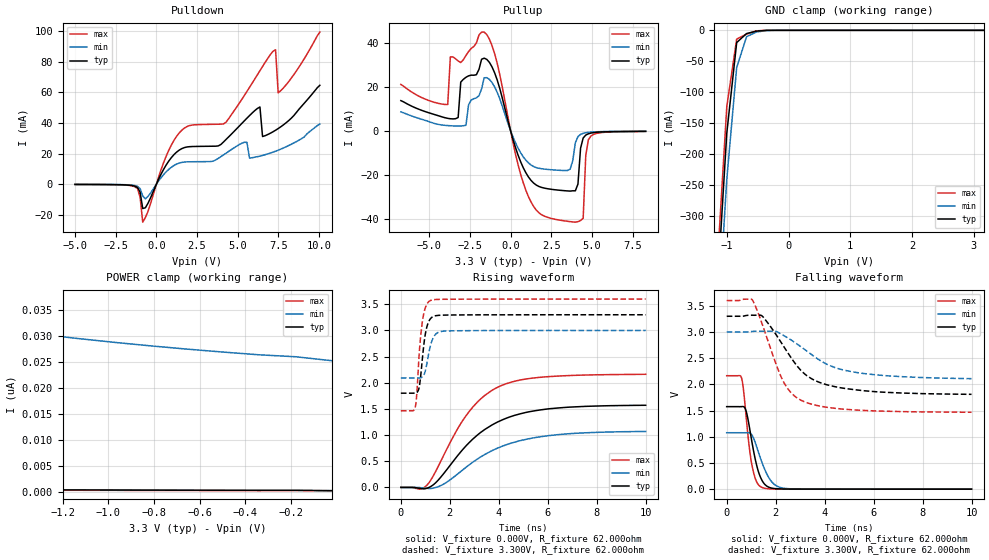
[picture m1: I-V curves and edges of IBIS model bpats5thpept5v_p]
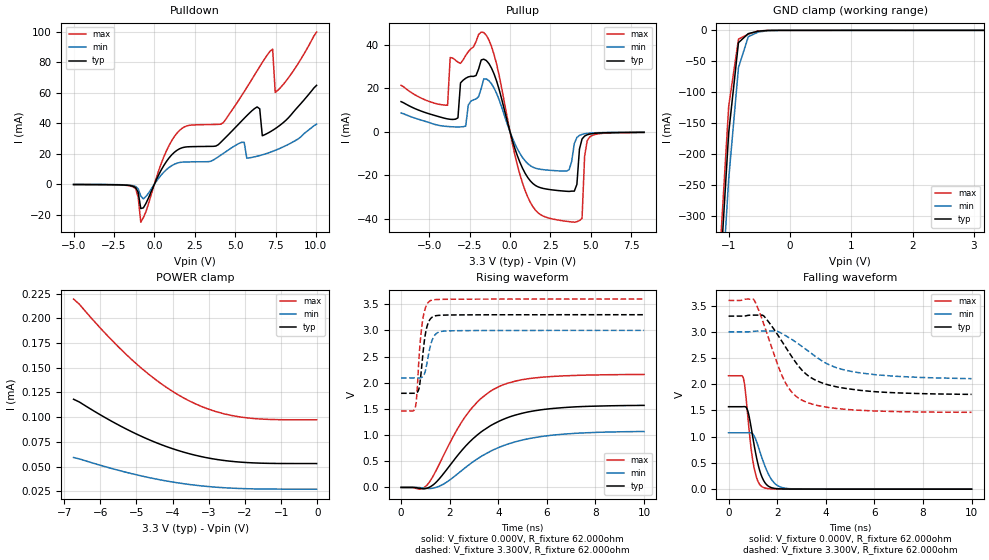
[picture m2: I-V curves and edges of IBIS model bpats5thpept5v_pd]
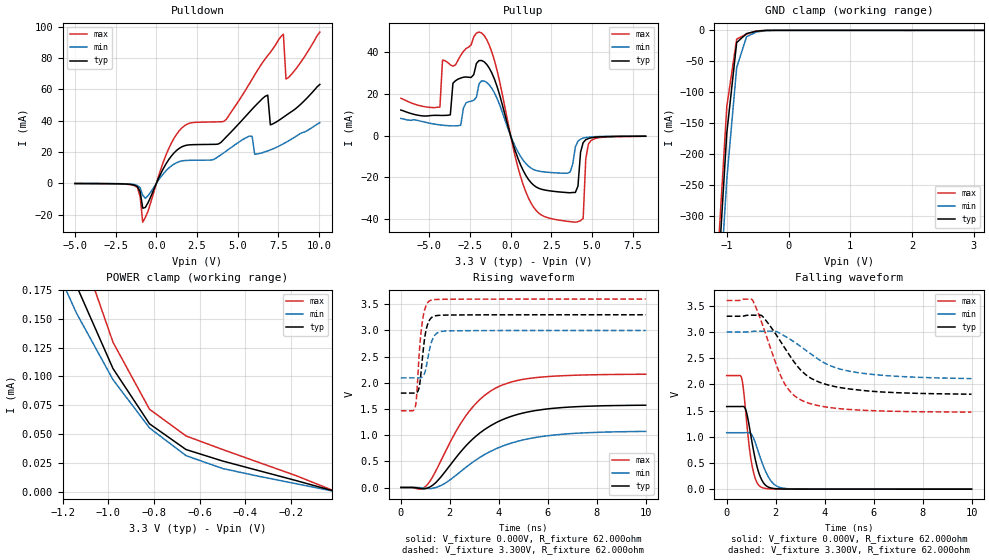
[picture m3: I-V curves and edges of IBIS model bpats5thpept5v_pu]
[IBIS Ver]  4.0
[File Name]  lpc176x.ibs
[File Rev]  1.0
[Date]   Tue Jul 28 17:01:21 PDT 2009
[Source]   Package model from Ansoft Q3D Extractor 7.1.1
[Notes]   IO models Rev 0.20 IBIS Model Design Automation Generation
[Copyright] NXP Semiconductors 2009. All rights reserved.
|   LPC1768 / 1766 / 1765 / 1764 IBIS Model
[Disclaimer]
| NXP Semiconductors warrants and represents that the IBIS models
| identified herein are owned by NXP Semiconductors (NXP).  The
| models provided are not warranted as fully representing all of the
| operating characteristics and specifications of the semiconductor
| products to which the models relate.  Moreover, unless there is a
| signed, written agreement to the contrary, these models are furnished
| on an "as is" basis without support or warranty of any kind, either
| expressed or implied, regarding the use thereof, and NXP
| specifically disclaims all implied warranties of merchantability and
| fitness of the models for any purpose.
| NXP does not assume any liability arising out of the application
| or use of these IBIS models including infringement of patents and
| copyrights, nor does NXP convey any license under its patents and
| copyrights or the rights of others.
| NXP provides IBIS models as a service to our customers.  You and
| your company shall not distribute, convey, sell, or give these models
| to anyone else without receiving prior written permission from
| NXP.
[Define Package Model]  LQFP100
[Manufacturer]  NXP Semiconductors
[OEM]  NXP
[Description]  LQFP100
|Sim freq : 100HMz
|Date : 7/28/09
[Number Of Pins]  100
[Pin Numbers]
1   | 1 = lead1
2   | 2 = lead2
3   | 3 = lead3
4   | 4 = lead4
5   | 5 = lead5
6   | 6 = lead6
7   | 7 = lead7
8   | 8 = lead8
9   | 9 = lead9
10   | 10 = lead10
11   | 11 = lead11
12   | 12 = lead12
13   | 13 = lead13
14   | 14 = lead14
15   | 15 = lead15
16   | 16 = lead16
17   | 17 = lead17
18   | 18 = lead18
19   | 19 = lead19
20   | 20 = lead20
21   | 21 = lead21
22   | 22 = lead22
23   | 23 = lead23
24   | 24 = lead24
25   | 25 = lead25
26   | 26 = lead26
27   | 27 = lead27
28   | 28 = lead28
29   | 29 = lead29
30   | 30 = lead30
31   | 31 = lead31
32   | 32 = lead32
33   | 33 = lead33
34   | 34 = lead34
35   | 35 = lead35
36   | 36 = lead36
37   | 37 = lead37
38   | 38 = lead38
39   | 39 = lead39
40   | 40 = lead40
41   | 41 = lead41
42   | 42 = lead42
43   | 43 = lead43
44   | 44 = lead44
45   | 45 = lead45
46   | 46 = lead46
47   | 47 = lead47
48   | 48 = lead48
49   | 49 = lead49
50   | 50 = lead50
51   | 51 = lead51
52   | 52 = lead52
53   | 53 = lead53
54   | 54 = lead54
55   | 55 = lead55
56   | 56 = lead56
57   | 57 = lead57
58   | 58 = lead58
59   | 59 = lead59
60   | 60 = lead60
61   | 61 = lead61
62   | 62 = lead62
63   | 63 = lead63
64   | 64 = lead64
65   | 65 = lead65
66   | 66 = lead66
67   | 67 = lead67
68   | 68 = lead68
69   | 69 = lead69
70   | 70 = lead70
71   | 71 = lead71
72   | 72 = lead72
73   | 73 = lead73
74   | 74 = lead74
75   | 75 = lead75
76   | 76 = lead76
77   | 77 = lead77
78   | 78 = lead78
79   | 79 = lead79
80   | 80 = lead80
81   | 81 = lead81
82   | 82 = lead82
83   | 83 = lead83
84   | 84 = lead84
85   | 85 = lead85
86   | 86 = lead86
87   | 87 = lead87
88   | 88 = lead88
89   | 89 = lead89
90   | 90 = lead90
91   | 91 = lead91
92   | 92 = lead92
93   | 93 = lead93
94   | 94 = lead94
95   | 95 = lead95
96   | 96 = lead96
97   | 97 = lead97
98   | 98 = lead98
99   | 99 = lead99
100   | 100 = lead100
[Model Data]
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[End Model Data]
[End Package Model]
[Component]   lpc176x
[Manufacturer]  NXP
[Package]
|   typ   min   max
R_pkg   0   0   0  |Values included in package model
L_pkg   0   0   0  |Values included in package model
C_pkg   0   0   0  |Values included in package model
[Package Model]  LQFP100
| (Pin and IO model definitions)
| IMPORTANT NOTES:
| The lpc176x GPIO pins, excluding the I2C and USB, have programmable input
| configurations. For this reason, three models are supplied for those basic
| padcells. Each model is identified by a unique suffix code at the end of
| the modelname:
| _p=plain input, _pd=pulldown enabled, _pu=pullup enabled
| The model_name for each of the GPIO pins in the [Pin] table below reflects
| the default state of that pin on power up (input with pullup enabled).
| The user may modify the model_name for a specific P#.# pin if that pin's
| input configuration is programmed differently from the default in the
| actual application. However, the model_names for all other pins are
| non-configurable and should not be altered.
| All GPIO padcells have 5ns slew rate control when operated as outputs,
| unless otherwise noted.
[Pin]   signal_name   model_name   | comments
1   TDO   bpts5ptpht5v_p   | 3-state output only
2   TDI   bpts5ptpht5v_pu   | In only
3   TMS   bpts5ptpht5v_pu   |
4   TRST_N   bpts5ptpht5v_pu   | In only
5   TCK   bpts5ptpht5v_p   | In only
6   P0.26   bpats5thpept5v_pu |
7   P0.25   bpats5thpept5v_pu |
8   P0.24   bpats5thpept5v_pu |
9   P0.23   bpats5thpept5v_pu |
10   VddA   POWER
11   VssA   GND
12   VREFP   POWER
13   Vdd   POWER
14   RSTOUTN   bpts5ptpht5v_pu   | Output only
15   VREFN   GND
16   RTCX1   NC
17   NRESET   bpts5ptpht5v_pu   | In only
18   RTCX2   NC
19   VBAT   POWER
20   P1.31   bpats5thpept5v_pu |
21   P1.30   bpats5thpept5v_pu |
22   X1   NC
23   X2   NC
24   P0.28   iic3m4sdat5v_400k | I2C padcell
25   P0.27   iic3m4sdat5v_400k | I2C padcell
26   P3.26   bpts5ptpht5v_pu   |
27   P3.25   bpts5ptpht5v_pu   |
28   Vdd   POWER
29   P0.29   usb11f1_iop_hs   | USB padcell
30   P0.30   usb11f1_iom_hs   | USB padcell
31   Vss   GND
32   P1.18   bpts5ptpht5v_pu   |
33   P1.19   bpts5ptpht5v_pu   |
34   P1.20   bpts5ptpht5v_pu   |
35   P1.21   bpts5ptpht5v_pu   |
36   P1.22   bpts5ptpht5v_pu   |
37   P1.23   bpts5ptpht5v_pu   |
38   P1.24   bpts5ptpht5v_pu   |
39   P1.25   bpts5ptpht5v_pu   |
40   P1.26   bpts5ptpht5v_pu   |
41   Vss   GND
42   Vdd   POWER
43   P1.27   bpts5ptpht5v_pu   |
44   P1.28   bpts5ptpht5v_pu   |
45   P1.29   bpts5ptpht5v_pu   |
46   P0.0   bpts5ptpht5v_pu   |
47   P0.1   bpts5ptpht5v_pu   |
48   P0.10   bpts5ptpht5v_pu   |
49   P0.11   bpts5ptpht5v_pu   |
50   P2.13   bpts5ptpht5v_pu   |
51   P2.12   bpts5ptpht5v_pu   |
52   P2.11   bpts5ptpht5v_pu   |
53   P2.10   bpts5ptpht5v_pu   |
54   Vdd   POWER
55   Vss   GND
56   P0.22   bpts5ptpht5v_pu   |
57   P0.21   bpts5ptpht5v_pu   |
58   P0.20   bpts5ptpht5v_pu   |
59   P0.19   bpts5ptpht5v_pu   |
60   P0.18   bpts5ptpht5v_pu   |
61   P0.17   bpts5ptpht5v_pu   |
62   P0.15   bpts5ptpht5v_pu   |
63   P0.16   bpts5ptpht5v_pu   |
64   P2.9   bpts5ptpht5v_pu   |
65   P2.8   bpts5ptpht5v_pu   |
66   P2.7   bpts5ptpht5v_pu   |
67   P2.6   bpts5ptpht5v_pu   |
68   P2.5   bpts5ptpht5v_pu   |
69   P2.4   bpts5ptpht5v_pu   |
70   P2.3   bpts5ptpht5v_pu   |
71   Vdd   POWER
72   Vss   GND
73   P2.2   bpts5ptpht5v_pu   |
74   P2.1   bpts5ptpht5v_pu   |
75   P2.0   bpts5ptpht5v_pu   |
76   P0.9   bpts5ptpht5v_pu   |
77   P0.8   bpts5ptpht5v_pu   |
78   P0.7   bpts5ptpht5v_pu   |
79   P0.6   bpts5ptpht5v_pu   |
80   P0.5   bpts5ptpht5v_pu   |
81   P0.4   bpts5ptpht5v_pu   |
82   P4.28   bpts5ptpht5v_pu   |
83   Vss   GND
84   Vdd   POWER
85   P4.29   bpts5ptpht5v_pu   |
86   P1.17   bpts5ptpht5v_pu   |
87   P1.16   bpts5ptpht5v_pu   |
88   P1.15   bpts5ptpht5v_pu   |
89   P1.14   bpts5ptpht5v_pu   |
90   P1.10   bpts5ptpht5v_pu   |
91   P1.9   bpts5ptpht5v_pu   |
92   P1.8   bpts5ptpht5v_pu   |
93   P1.4   bpts5ptpht5v_pu   |
94   P1.1   bpts5ptpht5v_pu   |
95   P1.0   bpts5ptpht5v_pu   |
96   Vdd   POWER
97   Vss   GND
98   P0.2   bpts5ptpht5v_pu   |
99   P0.3   bpts5ptpht5v_pu   |
100   RTCK   bpts5ptpht5v_pu   |
| Models and submodels in the file (9): bpats5thpept5v_p (I/O), bpats5thpept5v_pd (I/O), bpats5thpept5v_pu (I/O), bpts5ptpht5v_p (I/O), bpts5ptpht5v_pd (I/O), bpts5ptpht5v_pu (I/O), iic3m4sdat5v_400k (I/O_open_drain), usb11f1_iom_hs (I/O), usb11f1_iop_hs (I/O)
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| bpats5thpept5v
|   Bidirectional Pad 3v3
|   CMOS
|   Characterized at Core 1.8V and I/O 3.3V
| Plain input Mode (p1=0, p2=1)
[Model]   bpats5thpept5v_p | of bpats5thpept5v
Model_type   I/O
Polarity   Non-Inverting
Enable   Active-Low
|  Reciever Thresholds
Vinl   = 0.54V
Vinh   = 1.26V
| AC Test Load Conditions
Vref   = 0
Cref   = 1.2e-11
Rref   = 1000000000
Vmeas   = 0.9
| [Process Range]   typical   min   max
| C_comp edge width   400.000ps   400.000ps   400.000ps
| C_comp Tstrobe   40.000fs   40.000fs   40.000fs
C_comp   2.539pF   2.402pF   2.679pF
[Temperature Range]   25   125   -40
[Voltage Range]   3.30V   3.00V   3.60V
[GND Clamp Reference]   0.00V   0.00V   0.00V
[Pulldown Reference]   0.00V   0.00V   0.00V
[POWER Clamp Reference]   3.30V   3.00V   3.60V
[Pullup Reference]   3.30V   3.00V   3.60V
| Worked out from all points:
|   slope of the pulldown table from 0 to 0.495 V, typ, clamps not added: 46.5 ohm
|   slope of the pullup table from 0 to 0.495 V, typ, clamps not added: 41.9 ohm
|   GND clamp passes 1 mA (typ) near -0.48 V on its own axis
|   rising waveform, V_fixture 0.000V, R_fixture 62.000ohm: 20-80 % time 2.15ns typ, 2.37ns min, 1.8ns max; typ from 0 V to 1.57 V
|   falling waveform, V_fixture 0.000V, R_fixture 62.000ohm: 20-80 % time 411ps typ, 539ps min, 319ps max; typ from 1.57 V to 0 V
|   rising waveform, V_fixture 3.300V, R_fixture 62.000ohm: 20-80 % time 225ps typ, 260ps min, 215ps max; typ from 1.8 V to 3.3 V
|   falling waveform, V_fixture 3.300V, R_fixture 62.000ohm: 20-80 % time 1.53ns typ, 1.95ns min, 1.1ns max; typ from 3.3 V to 1.81 V
[GND Clamp]
| ref voltage   0.00V   0.00V   0.00V
|   Voltage   I(typ)   I(min)   I(max)
-5V       -7.933A    -7.953A    -7.929A
-1.16V    -429.6mA   -501mA     -389.4mA
-1V       -166.1mA   -240.8mA   -123.1mA
-840mV    -19.82mA   -60.19mA   -14.18mA
-680mV    -5.225mA   -10.28mA   -6.152mA
-520mV    -1.304mA   -2.7mA     -818.1uA
-200mV    -132.3nA   -9.731uA   -2.769nA
3.16V     216.3pA    26.32nA    148.8pA
[Power Clamp]   | Vtable = Vcc - Vpad
| ref voltage   3.30V   3.00V   3.60V
|   Voltage   I(typ)   I(min)   I(max)
-6.74V    1.379nA    125.5nA    723.8pA
-4.66V    863pA      70.57nA    560.5pA
-2.42V    509.5pA    38.28nA    388.3pA
-2.26V    489.9pA    36.89nA    376pA
-2.1V     470.8pA    35.59nA    363.8pA
-1.78V    434.1pA    33.27nA    339.4pA
-1.62V    416.5pA    32.24nA    327.2pA
-1.3V     382.5pA    30.41nA    302.8pA
-820mV    334.3pA    28.18nA    266.3pA
-340mV    288.9pA    26.43nA    229.9pA
-180mV    281.7pA    26.06nA    265.9pA
-20mV     233pA      25.29nA    176.8pA
[Pulldown]
| ref voltage   0.00V   0.00V   0.00V
|   Voltage   I(typ)   I(min)   I(max)
-5V       -187.5uA   -145.8uA   -211.8uA
-1.32V    -1.32mA    -939.5uA   -1.723mA
-1V       -5.324mA   -2.961mA   -8.618mA
-840mV    -15.95mA   -7.735mA   -24.89mA
1.4V      22.26mA    13.79mA    33.48mA
4.28V     29.27mA    20.27mA    40.55mA
5.56V     43.15mA    27.33mA    60.63mA
6.36V     50.49mA    18.36mA    74.24mA
6.52V     31.16mA    18.79mA    76.97mA
7.32V     35.27mA    21.55mA    87.95mA
7.48V     36.36mA    22.22mA    59.78mA
10.04V    64.68mA    39.32mA    99.49mA
[Pullup]   | Vtable = Vcc - Vpad
| ref voltage   3.30V   3.00V   3.60V
|   Voltage   I(typ)   I(min)   I(max)
-6.74V    13.67mA    8.53mA     21.02mA
-3.86V    5.598mA    2.307mA    11.88mA
-3.7V     5.416mA    2.227mA    33.56mA
-2.74V    24.29mA    2.441mA    34.22mA
-1.62V    32.99mA    24.07mA    44.83mA
940mV     -19.18mA   -13.46mA   -27.14mA
2.86V     -27.01mA   -17.98mA   -40.52mA
3.98V     -27.37mA   -5.511mA   -41.66mA
4.46V     -3.36mA    -1.235mA   -39.89mA
4.62V     -2.02mA    -961.6uA   -11.27mA
4.94V     -1.105mA   -662.3uA   -2.417mA
8.3V      -310.5uA   -276.1uA   -365.1uA
[Ramp]
R_load   = 62.000ohm
|   dV/dt(typ)   dV/dt(min)   dV/dt(max)
dV/dt_r   720.631mV/2.205ns   482.682mV/2.365ns   1.049V/2.035ns
dV/dt_f   674.653mV/1.565ns   397.637mV/1.940ns   1.038V/1.245ns
[Rising Waveform]  | cubic spline decimation from 2001 points
V_fixture   = 0.000V
R_fixture   = 62.000ohm
|   Time   V(typ)   V(min)   V(max)
0s        2.482nV    412.2nV    1.344nV
765ps     -17.12mV   -3.168mV   -33.52mV
1.06ns    -16.23mV   -17.53mV   40.55mV
1.715ns   244.2mV    54.65mV    580.5mV
2.665ns   795.4mV    385.7mV    1.372V
3.255ns   1.049V     581mV      1.689V
3.95ns    1.25V      750.6mV    1.914V
4.895ns   1.409V     895.8mV    2.055V
6.08ns    1.504V     991.8mV    2.119V
10ns      1.57V      1.07V      2.162V
[Falling Waveform]  | cubic spline decimation from 2001 points
V_fixture   = 0.000V
R_fixture   = 62.000ohm
|   Time   V(typ)   V(min)   V(max)
0s        1.575V     1.077V     2.165V
610ps     1.576V     1.077V     2.118V
680ps     1.576V     1.076V     1.921V
790ps     1.496V     1.077V     1.406V
1.025ns   917.9mV    1.038V     476.3mV
1.205ns   493mV      837.1mV    157.9mV
1.445ns   165.7mV    505.2mV    32.07mV
1.885ns   16.15mV    117.4mV    4.029mV
2.4ns     2.893mV    14.38mV    1.574mV
10ns      49.83uV    118.5uV    23.14uV
[Rising Waveform]  | cubic spline decimation from 2001 points
V_fixture   = 3.300V
V_fixture_min = 3.000V
V_fixture_max = 3.600V
R_fixture   = 62.000ohm
|   Time   V(typ)   V(min)   V(max)
0s        1.801V     2.092V     1.464V
585ps     1.801V     2.093V     1.532V
640ps     1.809V     2.093V     1.718V
755ps     1.929V     2.092V     2.589V
885ps     2.487V     2.116V     3.188V
1.03ns    3.005V     2.289V     3.47V
1.21ns    3.225V     2.71V      3.572V
1.41ns    3.281V     2.923V     3.591V
1.82ns    3.294V     2.989V     3.596V
10ns      3.3V       3V         3.6V
[Falling Waveform]  | cubic spline decimation from 2001 points
V_fixture   = 3.300V
V_fixture_min = 3.000V
V_fixture_max = 3.600V
R_fixture   = 62.000ohm
|   Time   V(typ)   V(min)   V(max)
0s        3.3V       3V         3.6V
1.04ns    3.32V      3.009V     3.616V
1.45ns    3.304V     3.014V     3.151V
2.045ns   2.929V     3.004V     2.35V
2.325ns   2.727V     2.933V     2.045V
2.66ns    2.488V     2.839V     1.826V
3.1ns     2.235V     2.695V     1.683V
4.145ns   1.986V     2.371V     1.559V
5.13ns    1.904V     2.24V      1.515V
10ns      1.81V      2.109V     1.468V
| bpats5thpept5v
|   Bidirectional Pad 3v3
|   CMOS
|   Characterized at Core 1.8V and I/O 3.3V
| Pull Down Mode (p1=1, p2=1)
[Model]   bpats5thpept5v_pd | of bpats5thpept5v
Model_type   I/O
Polarity   Non-Inverting
Enable   Active-Low
|  Reciever Thresholds
Vinl   = 0.54V
Vinh   = 1.26V
| AC Test Load Conditions
Vref   = 0
Cref   = 1.2e-11
Rref   = 1000000000
Vmeas   = 0.9
| [Process Range]   typical   min   max
| C_comp edge width   400.000ps   400.000ps   400.000ps
| C_comp Tstrobe   40.000fs   40.000fs   40.000fs
C_comp   2.538pF   2.399pF   2.678pF
[Temperature Range]   25   125   -40
[Voltage Range]   3.30V   3.00V   3.60V
[GND Clamp Reference]   0.00V   0.00V   0.00V
[Pulldown Reference]   0.00V   0.00V   0.00V
[POWER Clamp Reference]   3.30V   3.00V   3.60V
[Pullup Reference]   3.30V   3.00V   3.60V
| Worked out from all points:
|   slope of the pulldown table from 0 to 0.495 V, typ, clamps not added: 46.5 ohm
|   slope of the pullup table from 0 to 0.495 V, typ, clamps not added: 41.9 ohm
|   GND clamp passes 1 mA (typ) near -0.48 V on its own axis
|   rising waveform, V_fixture 0.000V, R_fixture 62.000ohm: 20-80 % time 2.15ns typ, 2.37ns min, 1.8ns max; typ from 0 V to 1.57 V
|   falling waveform, V_fixture 0.000V, R_fixture 62.000ohm: 20-80 % time 410ps typ, 538ps min, 318ps max; typ from 1.57 V to 0 V
|   rising waveform, V_fixture 3.300V, R_fixture 62.000ohm: 20-80 % time 227ps typ, 261ps min, 216ps max; typ from 1.8 V to 3.3 V
|   falling waveform, V_fixture 3.300V, R_fixture 62.000ohm: 20-80 % time 1.53ns typ, 1.95ns min, 1.1ns max; typ from 3.3 V to 1.81 V
[GND Clamp]
| ref voltage   0.00V   0.00V   0.00V
|   Voltage   I(typ)   I(min)   I(max)
-5V       -7.933A    -7.953A    -7.929A
-1.16V    -429.6mA   -501mA     -389.4mA
-1V       -166.1mA   -240.8mA   -123.1mA
-840mV    -19.84mA   -60.2mA    -14.2mA
-680mV    -5.244mA   -10.3mA    -6.181mA
-520mV    -1.329mA   -2.711mA   -860.7uA
-200mV    -17.4uA    -20.02uA   -26.89uA
3.16V     53.01uA    27.08uA    97.28uA
[Power Clamp]   | Vtable = Vcc - Vpad
| ref voltage   3.30V   3.00V   3.60V
|   Voltage   I(typ)   I(min)   I(max)
-6.74V    118.1uA    59.14uA    219.6uA
-6.58V    115.3uA    57.74uA    214.3uA
-6.1V     104.5uA    52.36uA    194.3uA
-5.62V    94.49uA    47.37uA    175.6uA
-4.98V    82.54uA    41.46uA    153.3uA
-4.5V     74.82uA    37.65uA    138.8uA
-4.18V    70.31uA    35.43uA    130.3uA
-3.54V    62.97uA    31.84uA    116.5uA
-2.9V     57.87uA    29.37uA    106.8uA
-2.1V     54.38uA    27.71uA    100uA
-1.3V     53.2uA     27.16uA    97.67uA
-20mV     53.01uA    27.08uA    97.29uA
[Pulldown]
| ref voltage   0.00V   0.00V   0.00V
|   Voltage   I(typ)   I(min)   I(max)
-5V       -187.5uA   -145.8uA   -211.8uA
-1.32V    -1.32mA    -939.5uA   -1.723mA
-1V       -5.324mA   -2.961mA   -8.619mA
-840mV    -15.95mA   -7.735mA   -24.89mA
1.4V      22.26mA    13.79mA    33.48mA
4.28V     29.29mA    20.29mA    40.56mA
5.56V     43.21mA    27.5mA     60.72mA
6.36V     50.67mA    18.36mA    74.36mA
6.68V     31.78mA    19.27mA    79.81mA
7.32V     35.33mA    21.55mA    88.56mA
7.48V     36.44mA    22.22mA    60.22mA
10.04V    64.83mA    39.4mA     99.75mA
[Pullup]   | Vtable = Vcc - Vpad
| ref voltage   3.30V   3.00V   3.60V
|   Voltage   I(typ)   I(min)   I(max)
-6.74V    13.82mA    8.599mA    21.35mA
-3.86V    5.864mA    2.372mA    12.19mA
-3.7V     5.685mA    2.288mA    34.11mA
-2.74V    24.57mA    2.531mA    35.04mA
-1.62V    33.35mA    24.26mA    45.59mA
940mV     -19.18mA   -13.46mA   -27.15mA
2.86V     -27.01mA   -17.98mA   -40.52mA
3.98V     -27.37mA   -5.511mA   -41.66mA
4.46V     -3.361mA   -1.235mA   -39.89mA
4.62V     -2.02mA    -961.6uA   -11.27mA
4.94V     -1.105mA   -662.3uA   -2.418mA
8.3V      -310.5uA   -276.1uA   -365.1uA
[Ramp]
R_load   = 62.000ohm
|   dV/dt(typ)   dV/dt(min)   dV/dt(max)
dV/dt_r   719.302mV/2.205ns   482.029mV/2.365ns   1.047V/2.040ns
dV/dt_f   675.416mV/1.570ns   397.994mV/1.940ns   1.039V/1.245ns
[Rising Waveform]  | cubic spline decimation from 2001 points
V_fixture   = 0.000V
R_fixture   = 62.000ohm
|   Time   V(typ)   V(min)   V(max)
0s        2.445nV    410.1nV    1.304nV
765ps     -17.11mV   -3.168mV   -33.47mV
1.06ns    -16.17mV   -17.52mV   40.67mV
1.685ns   226.6mV    47.31mV    550.5mV
2.675ns   798.3mV    388.8mV    1.374V
3.335ns   1.074V     602.8mV    1.717V
4.07ns    1.273V     772.5mV    1.936V
4.98ns    1.416V     903.8mV    2.058V
6.15ns    1.504V     994mV      2.117V
10ns      1.567V     1.068V     2.158V
[Falling Waveform]  | cubic spline decimation from 2001 points
V_fixture   = 0.000V
R_fixture   = 62.000ohm
|   Time   V(typ)   V(min)   V(max)
0s        1.572V     1.075V     2.162V
610ps     1.573V     1.075V     2.114V
680ps     1.573V     1.075V     1.917V
790ps     1.493V     1.076V     1.401V
1.025ns   915mV      1.036V     471.2mV
1.195ns   510.1mV    849.5mV    165.8mV
1.415ns   190.6mV    541.8mV    37.07mV
1.875ns   16.42mV    121.2mV    3.959mV
2.38ns    2.935mV    15.21mV    1.58mV
10ns      49.48uV    118uV      22.85uV
[Rising Waveform]  | cubic spline decimation from 2001 points
V_fixture   = 3.300V
V_fixture_min = 3.000V
V_fixture_max = 3.600V
R_fixture   = 62.000ohm
|   Time   V(typ)   V(min)   V(max)
0s        1.798V     2.091V     1.461V
590ps     1.799V     2.091V     1.537V
640ps     1.806V     2.091V     1.714V
755ps     1.926V     2.091V     2.583V
875ps     2.436V     2.11V      3.148V
1.015ns   2.967V     2.256V     3.446V
1.21ns    3.222V     2.708V     3.568V
1.415ns   3.279V     2.923V     3.588V
1.79ns    3.292V     2.987V     3.593V
10ns      3.299V     2.999V     3.598V
[Falling Waveform]  | cubic spline decimation from 2001 points
V_fixture   = 3.300V
V_fixture_min = 3.000V
V_fixture_max = 3.600V
R_fixture   = 62.000ohm
|   Time   V(typ)   V(min)   V(max)
0s        3.299V     2.999V     3.598V
1.035ns   3.318V     3.008V     3.614V
1.45ns    3.301V     3.013V     3.145V
2.005ns   2.954V     3.008V     2.395V
2.305ns   2.738V     2.937V     2.059V
2.63ns    2.506V     2.846V     1.835V
3.07ns    2.245V     2.704V     1.685V
4.13ns    1.985V     2.373V     1.556V
5.155ns   1.899V     2.236V     1.51V
10ns      1.807V     2.107V     1.465V
| bpats5thpept5v
|   Bidirectional Pad 3v3
|   CMOS
|   Characterized at Core 1.8V and I/O 3.3V
| Pull Up Mode (p1=0, p2=0)
[Model]   bpats5thpept5v_pu | of bpats5thpept5v
Model_type   I/O
Polarity   Non-Inverting
Enable   Active-Low
|  Reciever Thresholds
Vinl   = 0.54V
Vinh   = 1.26V
| AC Test Load Conditions
Vref   = 0
Cref   = 1.2e-11
Rref   = 1000000000
Vmeas   = 0.9
| [Process Range]   typical   min   max
| C_comp edge width   400.000ps   400.000ps   400.000ps
| C_comp Tstrobe   40.000fs   40.000fs   40.000fs
C_comp   2.536pF   2.398pF   2.677pF
[Temperature Range]   25   125   -40
[Voltage Range]   3.30V   3.00V   3.60V
[GND Clamp Reference]   0.00V   0.00V   0.00V
[Pulldown Reference]   0.00V   0.00V   0.00V
[POWER Clamp Reference]   3.30V   3.00V   3.60V
[Pullup Reference]   3.30V   3.00V   3.60V
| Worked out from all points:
|   slope of the pulldown table from 0 to 0.495 V, typ, clamps not added: 46.5 ohm
|   slope of the pullup table from 0 to 0.495 V, typ, clamps not added: 41.9 ohm
|   GND clamp passes 1 mA (typ) near -0.48 V on its own axis
|   POWER clamp passes 1 mA (typ) near -2.29 V on its own axis
|   rising waveform, V_fixture 0.000V, R_fixture 62.000ohm: 20-80 % time 2.14ns typ, 2.37ns min, 1.8ns max; typ from 0.001 V to 1.57 V
|   falling waveform, V_fixture 0.000V, R_fixture 62.000ohm: 20-80 % time 411ps typ, 539ps min, 320ps max; typ from 1.58 V to 0.001 V
|   rising waveform, V_fixture 3.300V, R_fixture 62.000ohm: 20-80 % time 224ps typ, 260ps min, 214ps max; typ from 1.8 V to 3.3 V
|   falling waveform, V_fixture 3.300V, R_fixture 62.000ohm: 20-80 % time 1.53ns typ, 1.95ns min, 1.1ns max; typ from 3.3 V to 1.81 V
[GND Clamp]
| ref voltage   0.00V   0.00V   0.00V
|   Voltage   I(typ)   I(min)   I(max)
-5V       -7.933A    -7.953A    -7.929A
-1.16V    -429.6mA   -501mA     -389.4mA
-1V       -166.1mA   -240.8mA   -123.1mA
-840mV    -19.83mA   -60.19mA   -14.19mA
-680mV    -5.242mA   -10.3mA    -6.178mA
-520mV    -1.331mA   -2.714mA   -864.2uA
-200mV    -50.25uA   -41.81uA   -77.56uA
3.16V     -7.353uA   6.327uA    -29.63uA
[Power Clamp]   | Vtable = Vcc - Vpad
| ref voltage   3.30V   3.00V   3.60V
|   Voltage   I(typ)   I(min)   I(max)
-6.74V    8.239mA    4.142mA    14.64mA
-1.3V     267.9uA    224.8uA    334.3uA
-1.14V    178.7uA    154.9uA    220.9uA
-980mV    106.8uA    97.21uA    129.7uA
-820mV    58.96uA    55.39uA    71.57uA
-660mV    36.65uA    31.38uA    48.44uA
-500mV    26.73uA    20.24uA    36.7uA
-180mV    9.891uA    7.111uA    14.19uA
-20mV     1.102uA    817.7nA    1.531uA
[Pulldown]
| ref voltage   0.00V   0.00V   0.00V
|   Voltage   I(typ)   I(min)   I(max)
-5V       -187.5uA   -145.8uA   -211.8uA
-1.32V    -1.32mA    -939.5uA   -1.723mA
-840mV    -15.95mA   -7.735mA   -24.89mA
1.56V     23.24mA    14.25mA    35.29mA
4.28V     29.46mA    20.48mA    40.61mA
5.72V     45.48mA    30.13mA    63.63mA
6.84V     56.23mA    20.64mA    81.58mA
7V        37.28mA    21.27mA    83.66mA
7.8V      42.14mA    25.2mA     95.19mA
7.96V     43.32mA    26.11mA    66.52mA
8.12V     44.49mA    27.07mA    67.59mA
10.04V    63.09mA    38.66mA    96.53mA
[Pullup]   | Vtable = Vcc - Vpad
| ref voltage   3.30V   3.00V   3.60V
|   Voltage   I(typ)   I(min)   I(max)
-6.74V    12.27mA    8.208mA    17.93mA
-4.34V    9.688mA    5.132mA    13.69mA
-4.18V    9.676mA    4.983mA    36.31mA
-3.06V    27.66mA    4.956mA    38.56mA
-1.78V    36.09mA    26.29mA    49.34mA
940mV     -19.18mA   -13.46mA   -27.14mA
3.02V     -27.13mA   -18.05mA   -40.73mA
3.98V     -27.37mA   -5.511mA   -41.66mA
4.46V     -3.361mA   -1.235mA   -39.89mA
4.62V     -2.02mA    -961.6uA   -11.27mA
4.94V     -1.105mA   -662.3uA   -2.418mA
8.3V      -310.5uA   -276.1uA   -365.1uA
[Ramp]
R_load   = 62.000ohm
|   dV/dt(typ)   dV/dt(min)   dV/dt(max)
dV/dt_r   721.276mV/2.205ns   483.044mV/2.365ns   1.050V/2.040ns
dV/dt_f   673.548mV/1.570ns   397.074mV/1.940ns   1.036V/1.245ns
[Rising Waveform]  | cubic spline decimation from 2001 points
V_fixture   = 0.000V
R_fixture   = 62.000ohm
|   Time   V(typ)   V(min)   V(max)
0s        1.219mV    1.008mV    1.479mV
765ps     -15.82mV   -2.159mV   -31.04mV
1.06ns    -13.88mV   -16.43mV   44.85mV
1.715ns   248mV      56.81mV    587.1mV
2.695ns   814.7mV    399.6mV    1.397V
3.235ns   1.045V     578mV      1.685V
3.985ns   1.261V     760.1mV    1.926V
4.8ns     1.401V     886.9mV    2.049V
5.97ns    1.501V     987.6mV    2.118V
10ns      1.572V     1.072V     2.164V
[Falling Waveform]  | cubic spline decimation from 2001 points
V_fixture   = 0.000V
R_fixture   = 62.000ohm
|   Time   V(typ)   V(min)   V(max)
0s        1.577V     1.078V     2.168V
605ps     1.578V     1.078V     2.128V
680ps     1.578V     1.078V     1.924V
790ps     1.499V     1.079V     1.41V
1.025ns   920.6mV    1.039V     480.1mV
1.21ns    485.9mV    831.8mV    153mV
1.415ns   193.6mV    545.1mV    38.94mV
1.845ns   19.81mV    137.4mV    6.125mV
2.33ns    4.655mV    18.77mV    3.371mV
10ns      1.272mV    1.133mV    1.504mV
[Rising Waveform]  | cubic spline decimation from 2001 points
V_fixture   = 3.300V
V_fixture_min = 3.000V
V_fixture_max = 3.600V
R_fixture   = 62.000ohm
|   Time   V(typ)   V(min)   V(max)
0s        1.804V     2.094V     1.467V
585ps     1.804V     2.094V     1.535V
640ps     1.811V     2.094V     1.722V
745ps     1.908V     2.094V     2.524V
880ps     2.466V     2.115V     3.176V
1.01ns    2.96V      2.249V     3.45V
1.2ns     3.219V     2.693V     3.573V
1.425ns   3.282V     2.93V      3.592V
1.755ns   3.293V     2.987V     3.596V
10ns      3.3V       3V         3.6V
[Falling Waveform]  | cubic spline decimation from 2001 points
V_fixture   = 3.300V
V_fixture_min = 3.000V
V_fixture_max = 3.600V
R_fixture   = 62.000ohm
|   Time   V(typ)   V(min)   V(max)
0s        3.3V       3V         3.6V
1.04ns    3.32V      3.009V     3.616V
1.45ns    3.304V     3.014V     3.152V
2.045ns   2.93V      3.004V     2.354V
2.325ns   2.728V     2.933V     2.048V
2.68ns    2.477V     2.833V     1.821V
3.07ns    2.251V     2.706V     1.693V
3.76ns    2.046V     2.474V     1.593V
4.99ns    1.914V     2.253V     1.522V
10ns      1.812V     2.11V      1.471V
